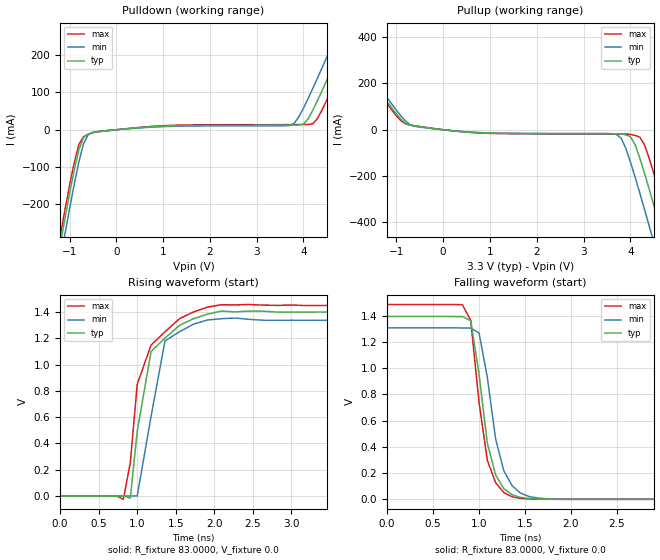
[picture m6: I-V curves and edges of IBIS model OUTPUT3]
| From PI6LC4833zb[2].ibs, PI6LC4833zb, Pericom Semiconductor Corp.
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|   Model OUTPUT3 (HCSL)
[Model]  OUTPUT3
Model_type Output
C_comp   5.5000pF   5.0000pF   6.0000pF
Vref = 0.00V
Vmeas = 0.35V
[Temperature Range]   25.0000   70.0000   -20
[Voltage Range]   3.3000V   3.1350V   3.4650V
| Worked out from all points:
|   slope of the pulldown table from 0 to 0.495 V, typ, clamps not added: 87.5 ohm
|   slope of the pullup table from 0 to 0.495 V, typ, clamps not added: 51.4 ohm
|   rising waveform, R_fixture 83.0000, V_fixture 0.0: 20-80 % time 247ps typ, 246ps min, 280ps max; typ from 0 V to 1.4 V
|   falling waveform, R_fixture 83.0000, V_fixture 0.0: 20-80 % time 182ps typ, 194ps min, 155ps max; typ from 1.39 V to 0 V
[Pulldown]
|Voltage   I(typ)   I(min)   I(max)
-3.3V     -1.864A    -1.903A    -1.842A
-1.2V     -309mA     -351.5mA   -285.8mA
-1.1V     -239mA     -281.1mA   -216.3mA
-800mV    -53.54mA   -86.05mA   -39.29mA
-700mV    -20.77mA   -37.28mA   -18.67mA
-500mV    -7.206mA   -6.909mA   -7.537mA
3.7V      12.34mA    11.24mA    13.71mA
4.2V      52.37mA    110.9mA    16.14mA
4.8V      218.8mA    281mA      164mA
5V        276.8mA    339.2mA    221.7mA
5.2V      335.4mA    397.7mA    280.1mA
6.6V      753.8mA    814.8mA    699mA
[Pullup]
|Voltage   I(typ)   I(min)   I(max)
-3.3V     730.8mA    746.6mA    722.2mA
-2.3V     437.8mA    454mA      428.8mA
-800mV    26.77mA    36.48mA    25.04mA
600mV     -11.15mA   -10.19mA   -11.93mA
3.7V      -17.37mA   -20.36mA   -18.45mA
4V        -30.01mA   -138mA     -19.92mA
4.2V      -120.7mA   -272mA     -31.84mA
4.4V      -254.8mA   -413.4mA   -121.8mA
4.5V      -325.2mA   -485.3mA   -187.7mA
4.7V      -469.1mA   -630.7mA   -327.8mA
4.9V      -615.2mA   -777.4mA   -472.4mA
6.6V      -1.881A    -2.043A    -1.737A
[Ramp]
| variable   typ   min   max
dV/dt_r  0.5146/77.3507p   0.4826/84.7389p   0.5491/78.8107p
dV/dt_f  0.3648/0.4177n   0.3144/0.4513n   0.4056/0.3997n
R_load = 50.0000
[Rising Waveform]
R_fixture= 83.0000
V_fixture= 0.0
|time   V(typ)   V(min)   V(max)
0s        0V         0V         0V
820ps     1.505mV    -7.234uV   -25.08mV
910ps     -16.18mV   17.71uV    254.3mV
1ns       495.1mV    1.217mV    851mV
1.18ns    1.101V     608.8mV    1.15V
1.36ns    1.203V     1.181V     1.25V
1.55ns    1.3V       1.251V     1.351V
1.91ns    1.384V     1.34V      1.438V
2.09ns    1.408V     1.35V      1.456V
9ns       1.397V     1.338V     1.448V
[Falling Waveform]
R_fixture= 83.0000
V_fixture= 0.0
|time   V(typ)   V(min)   V(max)
0s        1.393V     1.306V     1.484V
820ps     1.392V     1.305V     1.482V
910ps     1.361V     1.305V     1.362V
1ns       954.9mV    1.268V     740.7mV
1.09ns    430.4mV    932mV      297.7mV
1.18ns    187.5mV    462.6mV    127.9mV
1.27ns    80.44mV    216.6mV    50.82mV
1.36ns    35.1mV     104mV      19.3mV
1.82ns    291.5uV    1.489mV    -32.66uV
9ns       0V         0V         0V
